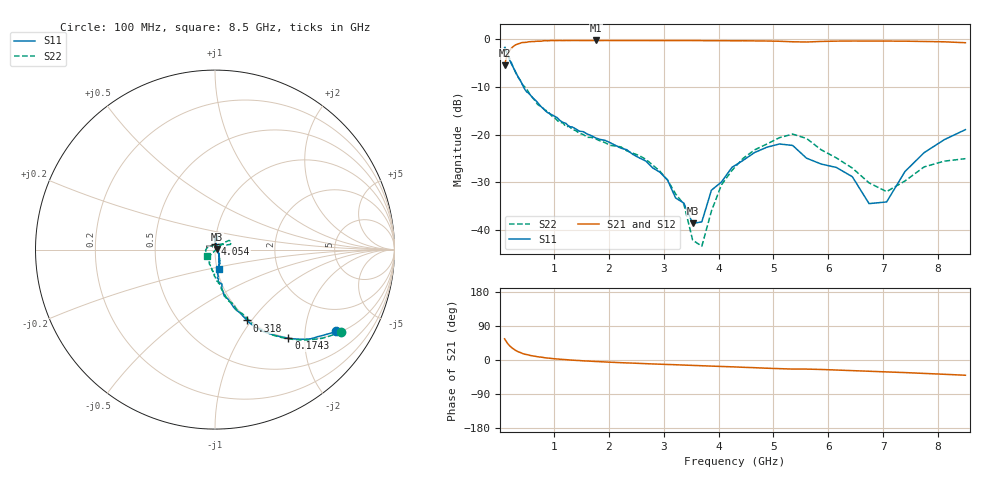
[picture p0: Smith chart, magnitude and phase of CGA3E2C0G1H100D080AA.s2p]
! S-parameter Generated by TDK Corporation
! Copyright(C) 2015 TDK Corporation.
! All Rights Reserved.
! TDK P/N: CGA3E2C0G1H100D080AA (Multilayer Ceramic Chip Capacitors)
! Property: C=10pF
! Size(LxWxT): 1.6x0.8x0.8mm, 0.063x0.031x0.031inches
! Model Type: s2p (Touchstone File Format Version 1.0)
! Frequency: DC=Yes Start=100MHz Stop=8500MHz 98points Log-sweep
! Note:
! Model Generated on Jun. 23, 2015
! Hash(MD5):
! Port Assignments:
!  1 ---| |--- 2
! Applicable Conditions:
!  Temperature = 25 degC
!  DC Bias Voltage = 0 V
!  Small Signal Operation
! Terms and conditions regarding TDK Simulation Models
! (1)This simulation model is being provided solely for informational purposes. Please refer to the specifications of the products in terms of detailed characteristics of such products.
! (2)In no event shall TDK Corporation of any of its subsidiaries be liable for any loss or damage arising, directly or indirectly,
!  From any information contained in this simulation model, including, but not limited to loss or damages arising from any inaccuracies, omissions or errors in connection with such information.
! (3)Any and all copyrights on this simulation model are owned by TDK Corporation.
!  Duplication or redistribution of this simulation model without prior written permission from TDK Corporation is prohibited.
! (4)This simulation model is subject to any modification or change without any prior notice.
! (5)Neither TDK Corporation nor any of its subsidiaries shall make any warranty, express or implied,
!  Including but not limited to the correctness, implied warranties of merchantability and fitness for a particular purpose with respect to this simulation models.
! (6)The use of this simulation model shall be deemed to have consented to the terms and conditions hereof.
# MHz S MA R 50
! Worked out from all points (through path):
!   97 points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, 100 MHz to 8.5 GHz, reference 50 ohm
!   highest |S21| = -0.25 dB at 1.762 GHz (marker M1); lowest = -5.5 dB at 100 MHz (marker M2)
!   group delay of S21, straight-line fit = 26.7 ps
!   lowest |S11| = -38.7 dB at 3.528 GHz (marker M3), VSWR 1.02, Z = 51.1 + j0.397 ohm
!   |S11| at or under -10 dB: 443.9 MHz to end of sweep
!   |S22| runs from -43.4 to -1.6 dB; largest |S21 - S12| = 0.0057
!   S11 on the Smith chart (normalised r, x): 100 MHz: 1.08, -2.91; 174.3 MHz: 0.99, -1.66; 318 MHz: 0.98, -0.95; 4.054 GHz: 1.00, +0.06; 8.5 GHz: 1.02, -0.23
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100  0.8137 -34.0  0.533 55.9  0.5323 55.9  0.8365 -33.1
174.2518  0.641 -50.4  0.7345 40.2  0.7331 40.2  0.6626 -49.0
318.0188  0.4338 -65.6  0.8828 24.0  0.8826 24.0  0.4259 -64.9
840.4526  0.1781 -84.2  0.9666 5.7  0.9671 5.7  0.1803 -84.5
1533.871  0.1073 -79.2  0.9699 -2.3  0.97 -2.2  0.1001 -102.1
1762.313  0.09207 -75.6  0.9718 -3.9  0.9711 -3.9  0.09012 -107.5
2931.989  0.04024 -56.6  0.9679 -11.1  0.9693 -11.1  0.04116 -130.7
3368.656  0.01904 -31.2  0.9699 -13.4  0.9689 -13.4  0.01852 -124.4
3528.213  0.01166 19.4  0.9694 -14.3  0.967 -14.2  0.007789 -101.5
3695.327  0.01214 42.7  0.9676 -15.2  0.9669 -15.2  0.006739 12.6
3870.357  0.02608 69.9  0.967 -16.1  0.9661 -16.0  0.01574 28.0
4053.677  0.03181 86.4  0.9668 -17.1  0.9661 -17.0  0.02974 34.5
4446.777  0.05356 92.7  0.9648 -19.2  0.9626 -19.1  0.05619 35.1
4877.997  0.0735 91.0  0.959 -21.7  0.9583 -21.6  0.07941 34.8
5351.035  0.07689 78.9  0.9413 -23.9  0.9416 -23.8  0.1011 27.2
5869.945  0.04905 90.3  0.9492 -25.0  0.9493 -24.9  0.06929 22.1
6439.175  0.03609 81.4  0.9589 -28.0  0.9587 -27.9  0.04447 42.6
6744.168  0.01884 52.7  0.9587 -29.7  0.9592 -29.6  0.03113 62.3
7063.606  0.01962 -22.3  0.9573 -31.4  0.9561 -31.3  0.02518 104.9
7398.175  0.04088 -56.2  0.9551 -33.2  0.954 -33.2  0.03256 145.5
7748.59  0.06466 -70.8  0.9482 -35.4  0.9518 -35.3  0.04578 167.4
8500  0.1126 -78.0  0.9202 -40.2  0.9226 -40.1  0.05585 -143.8
